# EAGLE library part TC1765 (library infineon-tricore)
TC1765 (AUDO1) 32-bit microcontroller for automotive and industrial applications (e.g. engine management, transmission, starter generator or 3-phase motor control) Source: http://www.infineon.com ..
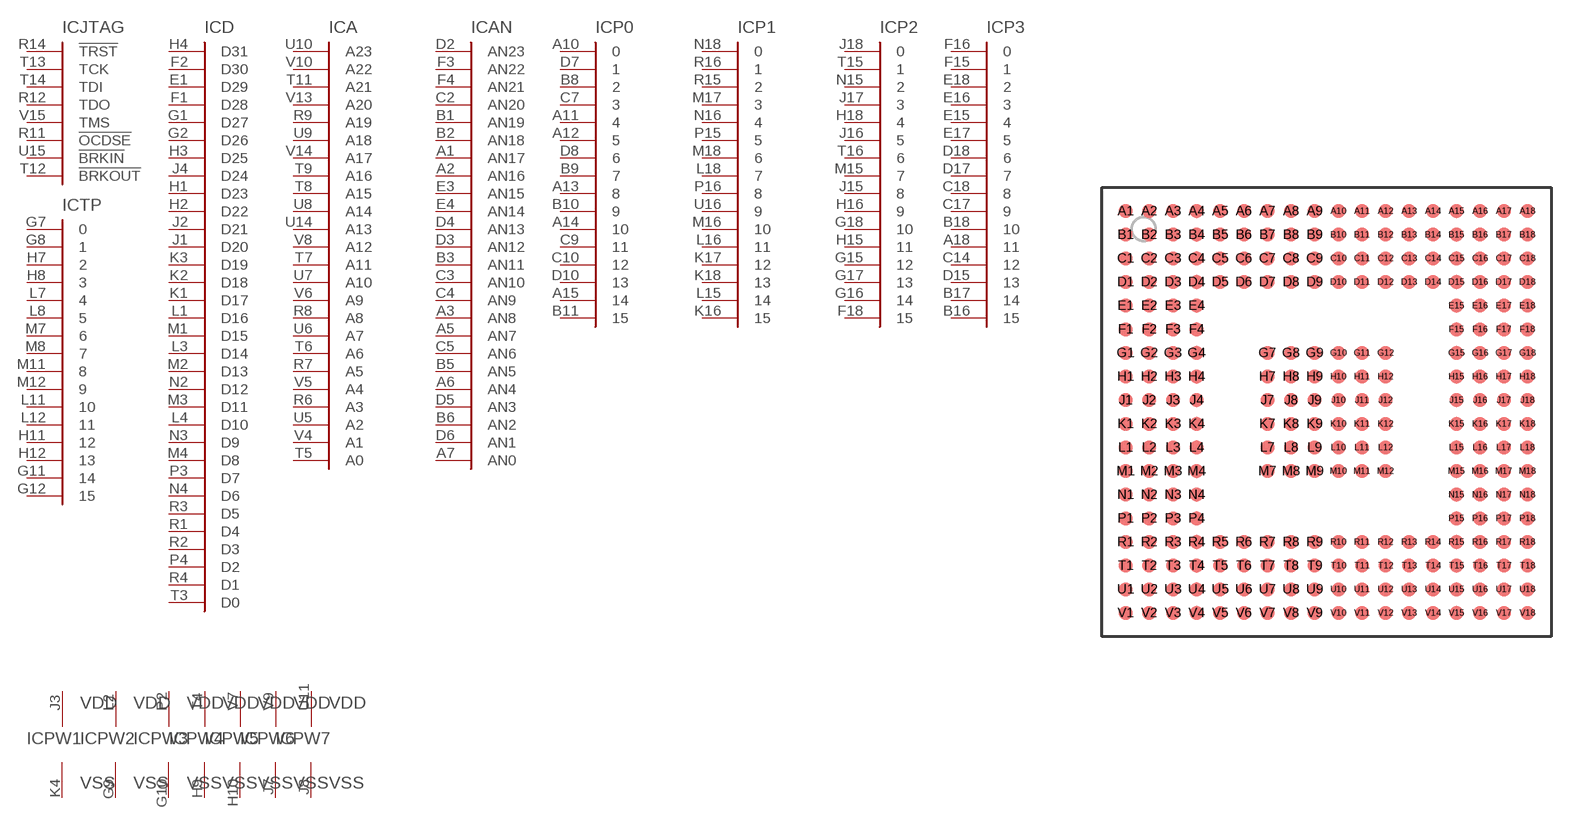
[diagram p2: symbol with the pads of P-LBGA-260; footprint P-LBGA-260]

Designator prefix IC; gates TP=PORT16 D=D31 A=A23 AN=AN23 JTAG=JTAG-OCSD P1=PORT16 P2=PORT16 P3=PORT16 P0=PORT16 PW1=VSS_VDD PW2=VSS_VDD PW3=VSS_VDD PW4=VSS_VDD PW5=VSS_VDD PW6=VSS_VDD PW7=VSS_VDD PW8=VSS_VDD PW9=VSS_VDD PW10=VSS_VDD G=TC1765 AREF0=VSS_VDD AREF1=VSS_VDD PW11=VSS_VDD PW12=VSS_VDD PW13=VSS_VDD PW14=VSS_VDD PW15=VSS_VDD PW16=VSS_VDD PW17=VSS_VDD PW18=VSS_VDD PW19=VSS_VDD PW20=VSS_VDD PW21=VSS_VDD PW23=GND6

## TC1765 (OC_FARNELL: unknown; OC_NEWARK: unknown)  [P-LBGA-260]
A1  AN:AN17  in
A2  AN:AN16  in
A3  AN:AN8  in
A4  PW11:VSS  pwr
A5  AN:AN7  in
A6  AN:AN4  in
A7  AN:AN0  in
A8  AREF1:VDD  pwr
A9  PW11:VDD  pwr
A10  P0:0  in
A11  P0:4  in
A12  P0:5  in
A13  P0:8  in
A14  P0:10  in
A15  P0:14  in
A16  G:P5.4
A17  G:P4.2
A18  P3:11  in
B1  AN:AN19  in
B2  AN:AN18  in
B3  AN:AN11  in
B4  PW12:VDD  pwr
B5  AN:AN5  in
B6  AN:AN2  in
B7  PW12:VSS  pwr
B8  P0:2  in
B9  P0:7  in
B10  P0:9  in
B11  P0:15  in
B12  PW13:VDD  pwr
B13  G:P5.1
B14  G:P5.2
B15  G:P4.3
B16  P3:15  in
B17  P3:14  in
B18  P3:10  in
C1  AREF0:VDD  pwr
C2  AN:AN20  in
C3  AN:AN10  in
C4  AN:AN9  in
C5  AN:AN6  in
C6  AREF1:VSS  pwr
C7  P0:3  in
C8  PW10:VDD  pwr
C9  P0:11  in
C10  P0:12  in
C11  G:P5.3
C12  G:P4.7
C13  G:P4.1
C14  P3:12  in
C15  G:P4.6
C16  G:P4.4
C17  P3:9  in
C18  P3:8  in
D1  PW13:VSS  pwr
D2  AN:AN23  in
D3  AN:AN12  in
D4  AN:AN13  in
D5  AN:AN3  in
D6  AN:AN1  in
D7  P0:1  in
D8  P0:6  in
D9  PW14:VSS  pwr
D10  P0:13  in
D11  PW14:VDD  pwr
D12  G:P5.0
D13  G:P4.5
D14  G:P4.0
D15  P3:13  in
D16  PW15:VDD  pwr
D17  P3:7  in
D18  P3:6  in
E1  D:D29
E2  AREF0:VSS  pwr
E3  AN:AN15  in
E4  AN:AN14  in
E15  P3:4  in
E16  P3:3  in
E17  P3:5  in
E18  P3:2  in
F1  D:D28
F2  D:D30
F3  AN:AN22  in
F4  AN:AN21  in
F15  P3:1  in
F16  P3:0  in
F17  PW9:VDD  pwr
F18  P2:15  in
G1  D:D27
G2  D:D26
G3  PW16:VDD  pwr
G4  PW17:VDD  pwr
G7  TP:0  in
G8  TP:1  in
G9  PW2:VSS  pwr
G10  PW3:VSS  pwr
G11  TP:14  in
G12  TP:15  in
G15  P2:12  in
G16  P2:14  in
G17  P2:13  in
G18  P2:10  in
H1  D:D23
H2  D:D22
H3  D:D25
H4  D:D31
H7  TP:2  in
H8  TP:3  in
H9  PW4:VSS  pwr
H10  PW5:VSS  pwr
H11  TP:12  in
H12  TP:13  in
H15  P2:11  in
H16  P2:9  in
H17  PW18:VDD  pwr
H18  P2:4  in
J1  D:D20
J2  D:D21
J3  PW1:VDD  pwr
J4  D:D24
J7  PW6:VSS  pwr
J8  PW7:VSS  pwr
J9  PW8:VSS  pwr
J10  PW9:VSS  pwr
J11  PW10:VSS  pwr
J12  PW15:VSS  pwr
J15  P2:8  in
J16  P2:5  in
J17  P2:3  in
J18  P2:0  in
K1  D:D17
K2  D:D18
K3  D:D19
K4  PW1:VSS  pwr
K7  PW16:VSS  pwr
K8  PW17:VSS  pwr
K9  PW18:VSS  pwr
K10  PW19:VSS  pwr
K11  PW20:VSS  pwr
K12  PW21:VSS  pwr
K15  PW23:GND  pwr
K16  P1:15  in
K17  P1:12  in
K18  P1:13  in
L1  D:D16
L2  PW2:VDD  pwr
L3  D:D14
L4  D:D10
L7  TP:4  in
L8  TP:5  in
L9  PW23:GND  pwr
L10  PW23:GND  pwr
L11  TP:10  in
L12  TP:11  in
L15  P1:14  in
L16  P1:11  in
L17  PW21:VDD  pwr
L18  P1:7  in
M1  D:D15
M2  D:D13
M3  D:D11
M4  D:D8
M7  TP:6  in
M8  TP:7  in
M9  PW23:GND  pwr
M10  PW23:GND  pwr
M11  TP:8  in
M12  TP:9  in
M15  P2:7  in
M16  P1:10  in
M17  P1:3  in
M18  P1:6  in
N1  G:ECIN
N2  D:D12
N3  D:D9
N4  D:D6
N15  P2:2  in
N16  P1:4  in
N17  G:BYPASS
N18  P1:0  in
P1  G:ECOUT
P2  PW3:VDD  pwr
P3  D:D7
P4  D:D2
P15  P1:5  in
P16  P1:8  in
P17  PW20:VDD  pwr
P18  G:/HDRST
R1  D:D4
R2  D:D3
R3  D:D5
R4  D:D1
R5  G:/WAIT/!IND
R6  A:A3  out
R7  A:A5  out
R8  A:A8  out
R9  A:A19  out
R10  G:/CS3
R11  JTAG:!OCDSE  in
R12  JTAG:TDO  out
R13  G:CPUCLK
R14  JTAG:!TRST  in
R15  P1:2  in
R16  P1:1  in
R17  PW23:GND  pwr
R18  PW19:VDD  pwr
T1  G:RD
T2  G:RD/!WR
T3  D:D0
T4  PW4:VDD  pwr
T5  A:A0  out
T6  A:A6  out
T7  A:A11  out
T8  A:A15  out
T9  A:A16  out
T10  G:/CS2
T11  A:A21  out
T12  JTAG:!BRKOUT  out
T13  JTAG:TCK  in
T14  JTAG:TDI  in
T15  P2:1  in
T16  P2:6  in
T17  G:/PO_RST
T18  G:XTAL2
U1  G:ADV
U2  G:/BC0
U3  G:/BC2
U4  G:/BAA
U5  A:A2  out
U6  A:A7  out
U7  A:A10  out
U8  A:A14  out
U9  A:A18  out
U10  A:A23  out
U11  PW7:VDD  pwr
U12  G:/CS0
U13  PW8:VDD  pwr
U14  A:A13  out
U15  JTAG:!BRKIN  in
U16  P1:9  in
U17  G:/NMI
U18  G:XTAL1
V1  G:/BC1
V2  G:/BC3
V3  G:/CODE
V4  A:A1  out
V5  A:A4  out
V6  A:A9  out
V7  PW5:VDD  pwr
V8  A:A12  out
V9  PW6:VDD  pwr
V10  A:A22  out
V11  G:/CDEMU/!CSOVK
V12  G:/CS1
V13  A:A20  out
V14  A:A17  out
V15  JTAG:TMS  in
V16  G:/TEST/MODE
V17  G:NC  nc
V18  G:NC  nc

## Footprint P-LBGA-260 (pad centres in mm)
P-LBGA-260 Plastic Ball Grid Array Package Source: http://www.infineon.com
smd 0.6 x 0.6: A1 -8.5,8.5; A2 -7.5,8.5; A3 -6.5,8.5; A4 -5.5,8.5; A5 -4.5,8.5; A6 -3.5,8.5; A7 -2.5,8.5; A8 -1.5,8.5; A9 -0.5,8.5; A10 0.5,8.5; A11 1.5,8.5; A12 2.5,8.5; A13 3.5,8.5; A14 4.5,8.5; A15 5.5,8.5; A16 6.5,8.5; A17 7.5,8.5; A18 8.5,8.5; B1 -8.5,7.5; B2 -7.5,7.5; B3 -6.5,7.5; B4 -5.5,7.5; B5 -4.5,7.5; B6 -3.5,7.5; B7 -2.5,7.5; B8 -1.5,7.5; B9 -0.5,7.5; B10 0.5,7.5; B11 1.5,7.5; B12 2.5,7.5; B13 3.5,7.5; B14 4.5,7.5; B15 5.5,7.5; B16 6.5,7.5; B17 7.5,7.5; B18 8.5,7.5; C1 -8.5,6.5; C2 -7.5,6.5; C3 -6.5,6.5; C4 -5.5,6.5; C5 -4.5,6.5; C6 -3.5,6.5; C7 -2.5,6.5; C8 -1.5,6.5; C9 -0.5,6.5; C10 0.5,6.5; C11 1.5,6.5; C12 2.5,6.5; C13 3.5,6.5; C14 4.5,6.5; C15 5.5,6.5; C16 6.5,6.5; C17 7.5,6.5; C18 8.5,6.5; D1 -8.5,5.5; D2 -7.5,5.5; D3 -6.5,5.5; D4 -5.5,5.5; D5 -4.5,5.5; D6 -3.5,5.5; D7 -2.5,5.5; D8 -1.5,5.5; D9 -0.5,5.5; D10 0.5,5.5; D11 1.5,5.5; D12 2.5,5.5; D13 3.5,5.5; D14 4.5,5.5; D15 5.5,5.5; D16 6.5,5.5; D17 7.5,5.5; D18 8.5,5.5; E1 -8.5,4.5; E2 -7.5,4.5; E3 -6.5,4.5; E4 -5.5,4.5; E15 5.5,4.5; E16 6.5,4.5; E17 7.5,4.5; E18 8.5,4.5; F1 -8.5,3.5; F2 -7.5,3.5; F3 -6.5,3.5; F4 -5.5,3.5; F15 5.5,3.5; F16 6.5,3.5; F17 7.5,3.5; F18 8.5,3.5; G1 -8.5,2.5; G2 -7.5,2.5; G3 -6.5,2.5; G4 -5.5,2.5; G7 -2.5,2.5; G8 -1.5,2.5; G9 -0.5,2.5; G10 0.5,2.5; G11 1.5,2.5; G12 2.5,2.5; G15 5.5,2.5; G16 6.5,2.5; G17 7.5,2.5; G18 8.5,2.5; H1 -8.5,1.5; H2 -7.5,1.5; H3 -6.5,1.5; H4 -5.5,1.5; H7 -2.5,1.5; H8 -1.5,1.5; H9 -0.5,1.5; H10 0.5,1.5; H11 1.5,1.5; H12 2.5,1.5; H15 5.5,1.5; H16 6.5,1.5; H17 7.5,1.5; H18 8.5,1.5; J1 -8.5,0.5; J2 -7.5,0.5; J3 -6.5,0.5; J4 -5.5,0.5; J7 -2.5,0.5; J8 -1.5,0.5; J9 -0.5,0.5; J10 0.5,0.5; J11 1.5,0.5; J12 2.5,0.5; J15 5.5,0.5; J16 6.5,0.5; J17 7.5,0.5; J18 8.5,0.5; K1 -8.5,-0.5; K2 -7.5,-0.5; K3 -6.5,-0.5; K4 -5.5,-0.5; K7 -2.5,-0.5; K8 -1.5,-0.5; K9 -0.5,-0.5; K10 0.5,-0.5; K11 1.5,-0.5; K12 2.5,-0.5; K15 5.5,-0.5; K16 6.5,-0.5; K17 7.5,-0.5; K18 8.5,-0.5; L1 -8.5,-1.5; L2 -7.5,-1.5; L3 -6.5,-1.5; L4 -5.5,-1.5; L7 -2.5,-1.5; L8 -1.5,-1.5; L9 -0.5,-1.5; L10 0.5,-1.5; L11 1.5,-1.5; L12 2.5,-1.5; L15 5.5,-1.5; L16 6.5,-1.5; L17 7.5,-1.5; L18 8.5,-1.5; M1 -8.5,-2.5; M2 -7.5,-2.5; M3 -6.5,-2.5; M4 -5.5,-2.5; M7 -2.5,-2.5; M8 -1.5,-2.5; M9 -0.5,-2.5; M10 0.5,-2.5; M11 1.5,-2.5; M12 2.5,-2.5; M15 5.5,-2.5; M16 6.5,-2.5; M17 7.5,-2.5; M18 8.5,-2.5; N1 -8.5,-3.5; N2 -7.5,-3.5; N3 -6.5,-3.5; N4 -5.5,-3.5; N15 5.5,-3.5; N16 6.5,-3.5; N17 7.5,-3.5; N18 8.5,-3.5; P1 -8.5,-4.5; P2 -7.5,-4.5; P3 -6.5,-4.5; P4 -5.5,-4.5; P15 5.5,-4.5; P16 6.5,-4.5; P17 7.5,-4.5; P18 8.5,-4.5; R1 -8.5,-5.5; R2 -7.5,-5.5; R3 -6.5,-5.5; R4 -5.5,-5.5; R5 -4.5,-5.5; R6 -3.5,-5.5; R7 -2.5,-5.5; R8 -1.5,-5.5; R9 -0.5,-5.5; R10 0.5,-5.5; R11 1.5,-5.5; R12 2.5,-5.5; R13 3.5,-5.5; R14 4.5,-5.5; R15 5.5,-5.5; R16 6.5,-5.5; R17 7.5,-5.5; R18 8.5,-5.5; T1 -8.5,-6.5; T2 -7.5,-6.5; T3 -6.5,-6.5; T4 -5.5,-6.5; T5 -4.5,-6.5; T6 -3.5,-6.5; T7 -2.5,-6.5; T8 -1.5,-6.5; T9 -0.5,-6.5; T10 0.5,-6.5; T11 1.5,-6.5; T12 2.5,-6.5; T13 3.5,-6.5; T14 4.5,-6.5; T15 5.5,-6.5; T16 6.5,-6.5; T17 7.5,-6.5; T18 8.5,-6.5; U1 -8.5,-7.5; U2 -7.5,-7.5; U3 -6.5,-7.5; U4 -5.5,-7.5; U5 -4.5,-7.5; U6 -3.5,-7.5; U7 -2.5,-7.5; U8 -1.5,-7.5; U9 -0.5,-7.5; U10 0.5,-7.5; U11 1.5,-7.5; U12 2.5,-7.5; U13 3.5,-7.5; U14 4.5,-7.5; U15 5.5,-7.5; U16 6.5,-7.5; U17 7.5,-7.5; U18 8.5,-7.5; V1 -8.5,-8.5; V2 -7.5,-8.5; V3 -6.5,-8.5; V4 -5.5,-8.5; V5 -4.5,-8.5; V6 -3.5,-8.5; V7 -2.5,-8.5; V8 -1.5,-8.5; V9 -0.5,-8.5; V10 0.5,-8.5; V11 1.5,-8.5; V12 2.5,-8.5; V13 3.5,-8.5; V14 4.5,-8.5; V15 5.5,-8.5; V16 6.5,-8.5; V17 7.5,-8.5; V18 8.5,-8.5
